(* Logix 5000 AddOnInstructionDefinition export YAI_Assy_151_101_EIP_Hz; software revision 17.00 *)

ADD_ON_INSTRUCTION YAI_Assy_151_101_EIP_Hz   (* revision 1.0, vendor Yaskawa America, Inc. *)
// YAI Assembly 151 and 101
// Help:
// This add-on instruction is for use with input assemblie 151 and output assemblies 101.
// Node_Input_Assy is defined as the node's input assembly integer array.
// Node_Output_Assy is defined as the node's output assembly integer array.
// Torque limit/reference, torque compensation and torque output variables are only available with A1000.
VAR_IN_OUT
   Node_Input_Assy : AB:ETHERNET_MODULE_INT_8Bytes:I:0; {required}   // Input assembly words
   Node_Output_Assy : AB:ETHERNET_MODULE_INT_8Bytes:O:0; {required}   // Output assembly words
END_VAR
VAR_INPUT
   RunFwd : BOOL; {visible}   // Forward run command
   RunRev : BOOL; {visible}   // Reverse run command
   MFI_3 : BOOL; {visible}   // Multi-function input 3
   MFI_4 : BOOL; {visible}   // Multi-function input 4
   MFI_5 : BOOL; {visible}   // Multi-function input 5
   MFI_6 : BOOL; {visible}   // Multi-function input 6
   MFI_7 : BOOL; {visible}   // Multi-function input 7
   MFI_8 : BOOL; {visible}   // Multi-function input 8
   External_Fault : BOOL;   // External fault command (EF0)
   FaultReset : BOOL; {visible}   // Fault reset command
   MFO_1 : BOOL; {visible}   // Multi-function output (M1-M2 for A/P1000, MA/MB/MC for V1000)
   MFO_2 : BOOL; {visible}   // Multi-function output (M3-M4 for A/P1000, P1 for V1000)
   MFO_3 : BOOL; {visible}   // Multi-function output (M5-M6 for A/P1000, P2 for V1000)
   Freq_Ref : REAL; {visible}   // Frequency reference command in Hz (xx.xx resolution)
   Torq_Ref_Limit : REAL; {visible}   // Torque reference/limit (A1000 only)
   Torq_Comp : REAL; {visible}   // Torque compensation command (A1000 only)
END_VAR
VAR_OUTPUT
   Running : BOOL; {visible}   // Drive running forward status bit
   ZSP : BOOL; {visible}   // Drive zero speed status bit
   RunningRev : BOOL; {visible}   // Drive running reverse status bit
   Reset : BOOL; {visible}   // Drive reset command status bit
   At_Speed : BOOL; {visible}   // Drive at commanded speed status bit
   Ready : BOOL; {visible}   // Drive ready status bit
   Alarm : BOOL; {visible}   // Drive alarm status bit
   Faulted : BOOL; {visible}   // Drive faulted status bit
   OPE : BOOL;   // OPE alarm/fault present
   UV : BOOL;   // Drive in UV (undervoltage) state status bit
   NetCtrlStatus : BOOL; {visible}   // Drive network run source status bit (1 = source coming from network)
   MFO_1_Status : BOOL; {visible}   // Drive multi-function output 1 (M1-M2 for A/P1000, MA/MB/MC for V1000) status
   MFO_2_Status : BOOL; {visible}   // Drive multi-function output 1 (M3-M4 for A/P1000, P1 for V1000) status
   MFO_3_Status : BOOL; {visible}   // Drive multi-function output 1 (M5-M6 for A/P1000, P2 for V1000) status
   ZSV : BOOL; {visible}   // Drive zero servo completed status bit
   Output_Freq : REAL; {visible}   // Drive output frequency in Hz (xx.xx resolution)
END_VAR
VAR_INPUT
   Torque_Actual : REAL; {visible}   // Drive torque output in % (xxx.x resolution)
   Output_Current : REAL; {visible}   // Drive output current in A (xxx.x resolution)
END_VAR
VAR
   FRef_Convert : DINT;
   FOut_Convert : REAL;
   FOut_Temp : REAL;
   TRef_Convert : INT;
   TComp_Convert : INT;
   TOut_Convert : REAL;
   TOut_Temp : REAL;
   IOut_Temp : REAL;
   IOut_Convert : REAL;
END_VAR

ROUTINE Logic   (* ladder *)
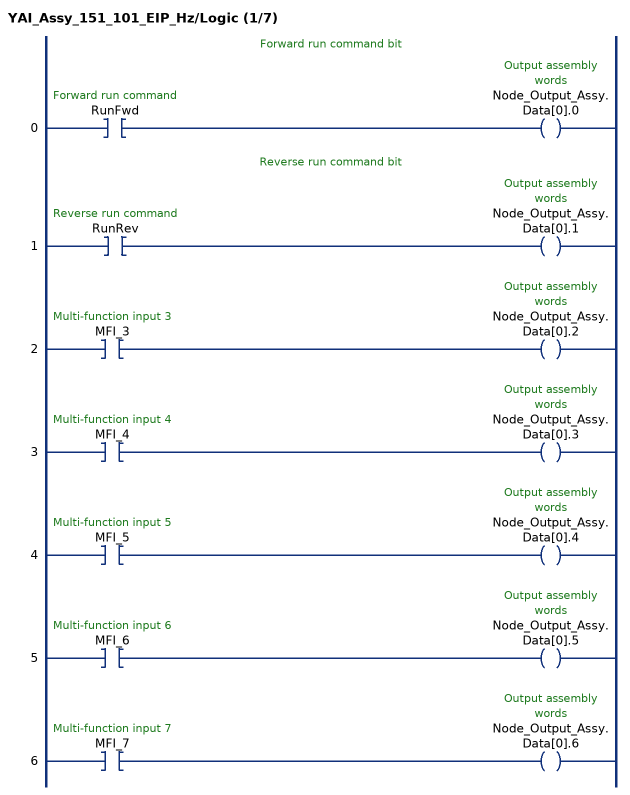
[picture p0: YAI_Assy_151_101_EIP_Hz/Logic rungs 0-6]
   // Forward run command bit
   0: XIC(RunFwd)OTE(Node_Output_Assy.Data[0].0);
   // Reverse run command bit
   1: XIC(RunRev)OTE(Node_Output_Assy.Data[0].1);
   2: XIC(MFI_3)OTE(Node_Output_Assy.Data[0].2);
   3: XIC(MFI_4)OTE(Node_Output_Assy.Data[0].3);
   4: XIC(MFI_5)OTE(Node_Output_Assy.Data[0].4);
   5: XIC(MFI_6)OTE(Node_Output_Assy.Data[0].5);
   6: XIC(MFI_7)OTE(Node_Output_Assy.Data[0].6);
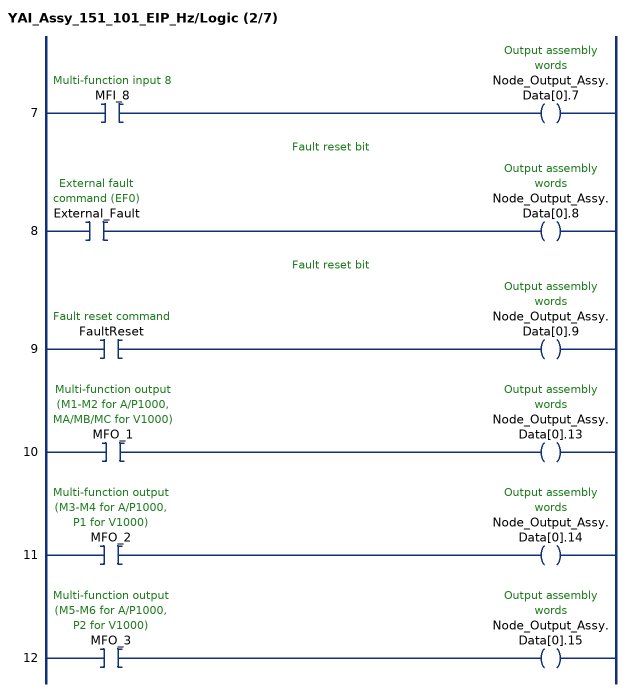
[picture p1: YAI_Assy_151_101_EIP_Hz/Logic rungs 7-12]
   7: XIC(MFI_8)OTE(Node_Output_Assy.Data[0].7);
   // Fault reset bit
   8: XIC(External_Fault)OTE(Node_Output_Assy.Data[0].8);
   // Fault reset bit
   9: XIC(FaultReset)OTE(Node_Output_Assy.Data[0].9);
   10: XIC(MFO_1)OTE(Node_Output_Assy.Data[0].13);
   11: XIC(MFO_2)OTE(Node_Output_Assy.Data[0].14);
   12: XIC(MFO_3)OTE(Node_Output_Assy.Data[0].15);
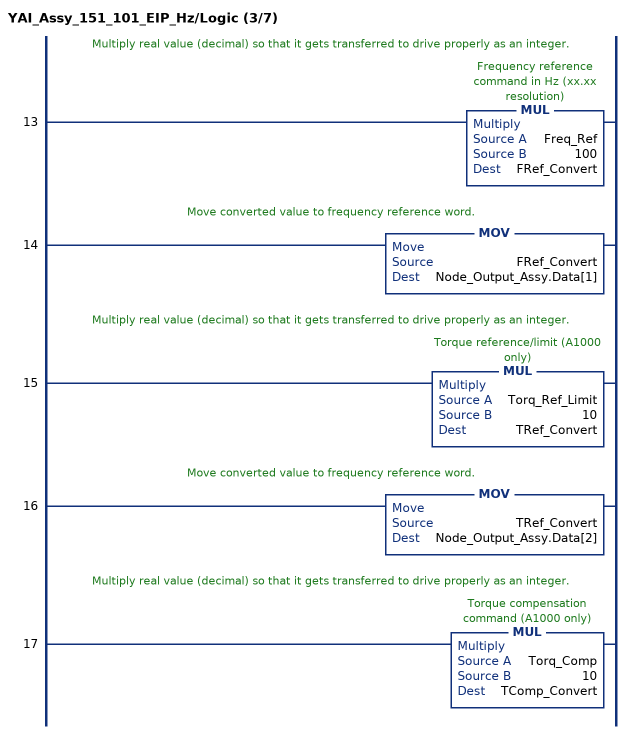
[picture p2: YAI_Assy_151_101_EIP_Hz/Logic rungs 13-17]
   // Multiply real value (decimal) so that it gets transferred to drive properly as an integer.
   13: MUL(Freq_Ref,100,FRef_Convert);
   // Move converted value to frequency reference word.
   14: MOV(FRef_Convert,Node_Output_Assy.Data[1]);
   // Multiply real value (decimal) so that it gets transferred to drive properly as an integer.
   15: MUL(Torq_Ref_Limit,10,TRef_Convert);
   // Move converted value to frequency reference word.
   16: MOV(TRef_Convert,Node_Output_Assy.Data[2]);
   // Multiply real value (decimal) so that it gets transferred to drive properly as an integer.
   17: MUL(Torq_Comp,10,TComp_Convert);
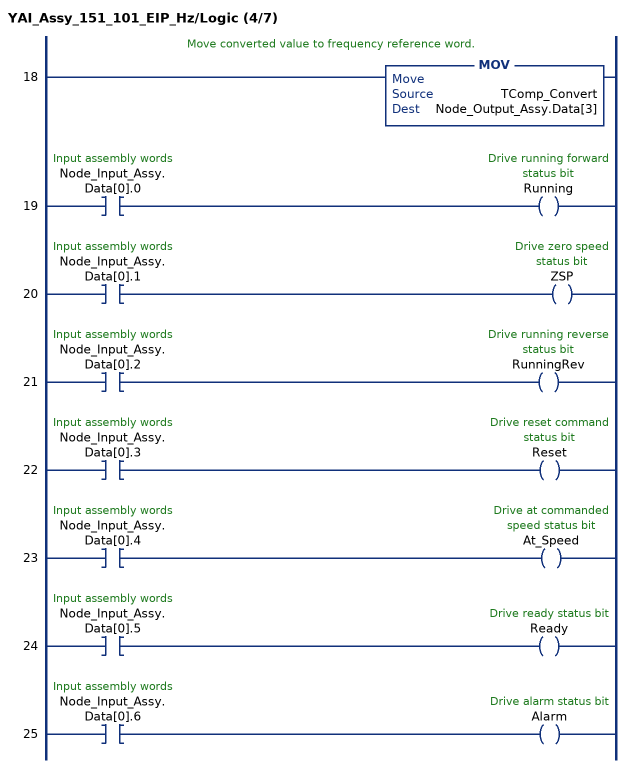
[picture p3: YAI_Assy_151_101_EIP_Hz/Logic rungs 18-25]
   // Move converted value to frequency reference word.
   18: MOV(TComp_Convert,Node_Output_Assy.Data[3]);
   19: XIC(Node_Input_Assy.Data[0].0)OTE(Running);
   20: XIC(Node_Input_Assy.Data[0].1)OTE(ZSP);
   21: XIC(Node_Input_Assy.Data[0].2)OTE(RunningRev);
   22: XIC(Node_Input_Assy.Data[0].3)OTE(Reset);
   23: XIC(Node_Input_Assy.Data[0].4)OTE(At_Speed);
   24: XIC(Node_Input_Assy.Data[0].5)OTE(Ready);
   25: XIC(Node_Input_Assy.Data[0].6)OTE(Alarm);
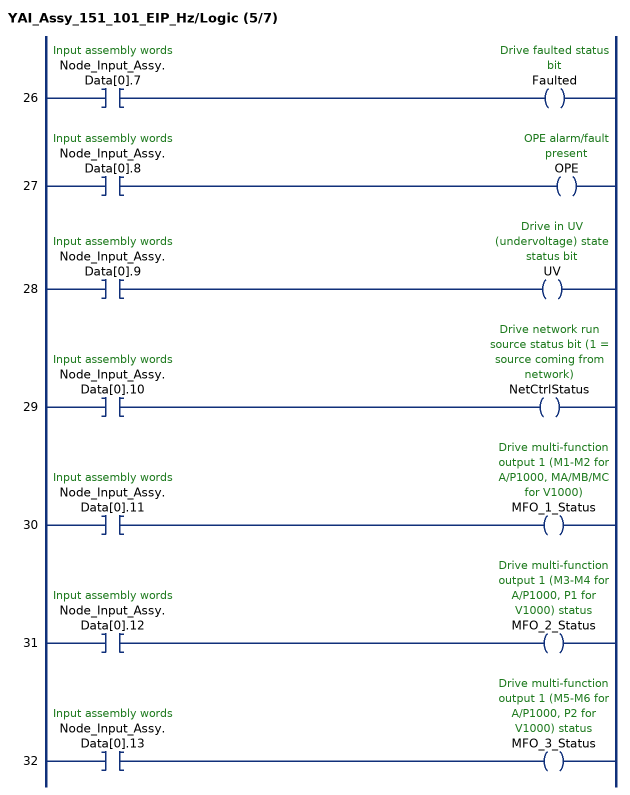
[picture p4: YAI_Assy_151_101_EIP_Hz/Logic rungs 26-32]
   26: XIC(Node_Input_Assy.Data[0].7)OTE(Faulted);
   27: XIC(Node_Input_Assy.Data[0].8)OTE(OPE);
   28: XIC(Node_Input_Assy.Data[0].9)OTE(UV);
   29: XIC(Node_Input_Assy.Data[0].10)OTE(NetCtrlStatus);
   30: XIC(Node_Input_Assy.Data[0].11)OTE(MFO_1_Status);
   31: XIC(Node_Input_Assy.Data[0].12)OTE(MFO_2_Status);
   32: XIC(Node_Input_Assy.Data[0].13)OTE(MFO_3_Status);
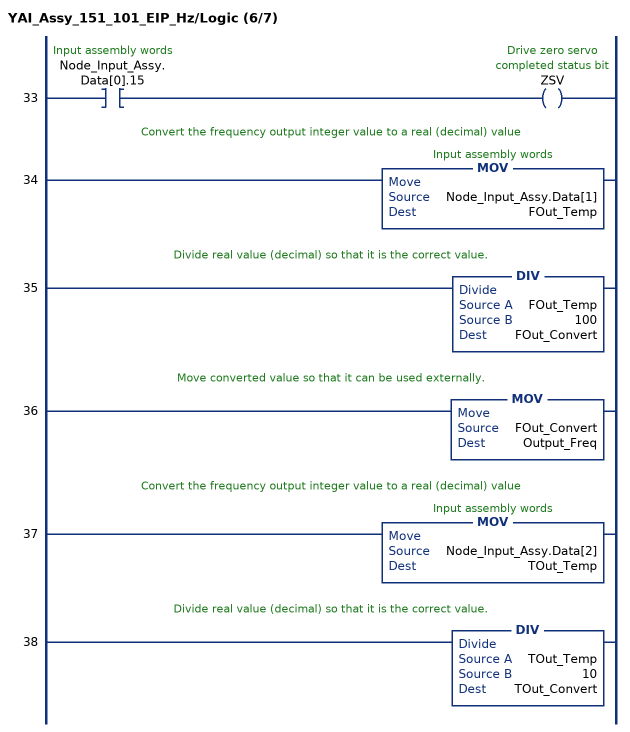
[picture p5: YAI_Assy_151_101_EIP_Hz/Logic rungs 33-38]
   33: XIC(Node_Input_Assy.Data[0].15)OTE(ZSV);
   // Convert the frequency output integer value to a real (decimal) value
   34: MOV(Node_Input_Assy.Data[1],FOut_Temp);
   // Divide real value (decimal) so that it is the correct value.
   35: DIV(FOut_Temp,100,FOut_Convert);
   // Move converted value so that it can be used externally.
   36: MOV(FOut_Convert,Output_Freq);
   // Convert the frequency output integer value to a real (decimal) value
   37: MOV(Node_Input_Assy.Data[2],TOut_Temp);
   // Divide real value (decimal) so that it is the correct value.
   38: DIV(TOut_Temp,10,TOut_Convert);
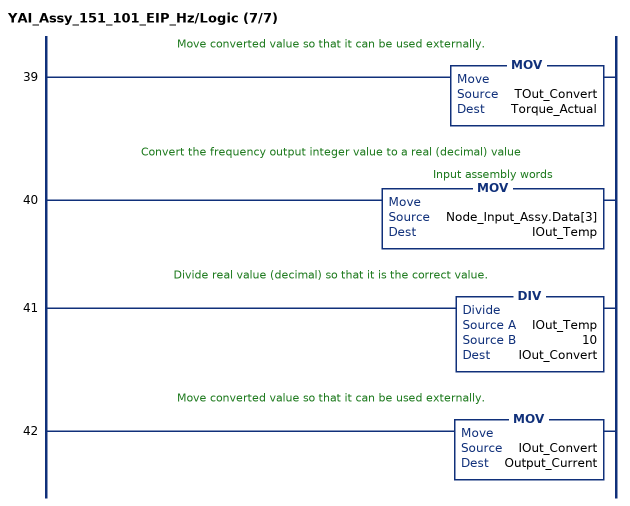
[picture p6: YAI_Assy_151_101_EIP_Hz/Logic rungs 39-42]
   // Move converted value so that it can be used externally.
   39: MOV(TOut_Convert,Torque_Actual);
   // Convert the frequency output integer value to a real (decimal) value
   40: MOV(Node_Input_Assy.Data[3],IOut_Temp);
   // Divide real value (decimal) so that it is the correct value.
   41: DIV(IOut_Temp,10,IOut_Convert);
   // Move converted value so that it can be used externally.
   42: MOV(IOut_Convert,Output_Current);
END_ROUTINE
END_ADD_ON_INSTRUCTION
